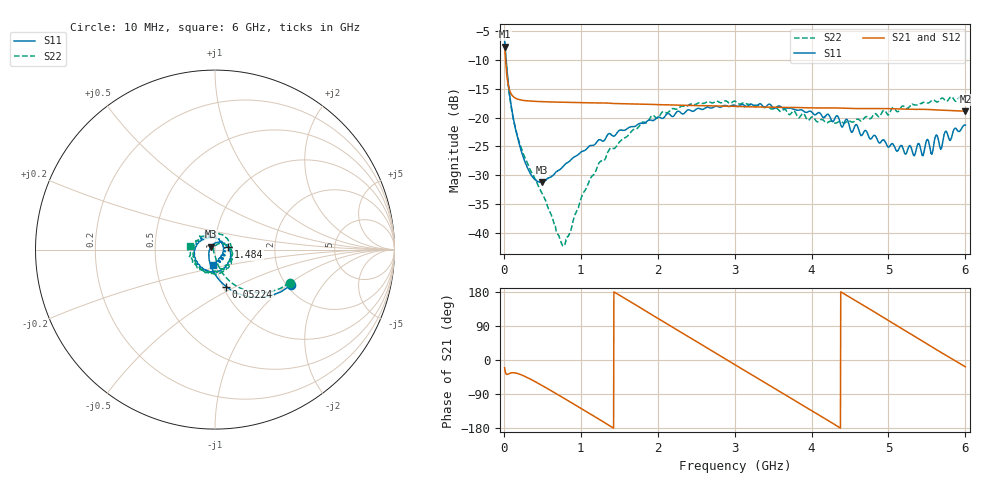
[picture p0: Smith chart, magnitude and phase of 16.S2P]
!Agilent Technologies,E5071C,MY46316741,A.11.02
!Date: Thu Jul 30 16:13:29 2020
!Data & Calibration Information:
!Freq	S11:SOLT4(ON)	S21:SOLT4(ON)	S12:SOLT4(ON)	S22:SOLT4(ON)
!PortZ  Port1:50+j0  Port2:50+j0
!Above PortZ is port z conversion or system Z0 setting when saving the data.
!When reading, reference impedance value at option line is always used.
# Hz S dB R 50
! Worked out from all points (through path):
!   1561 points, 10 MHz to 6 GHz, reference 50 ohm
!   highest |S21| = -7.68 dB at 10 MHz (marker M1); lowest = -18.9 dB at 6 GHz (marker M2)
!   group delay of S21, straight-line fit = 337 ps
!   lowest |S11| = -31.2 dB at 493.8 MHz (marker M3), VSWR 1.06, Z = 47.8 + j1.56 ohm
!   |S11| at or under -10 dB: 29.81 MHz to end of sweep
!   |S22| runs from -42.3 to -6.8 dB; largest |S21 - S12| = 0.0019
!   S11 on the Smith chart (normalised r, x): 10 MHz: 2.10, -1.07; 52.24 MHz: 1.03, -0.45; 1.484 GHz: 1.16, +0.03; 6 GHz: 0.96, -0.16
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1e7  -6.61 -25.1  -7.68 -20.5  -7.68 -20.5  -6.85 -23.9
5.223718e7  -13.35 -73.2  -13.96 -37.4  -13.96 -37.4  -13.71 -63.4
1.290321e8  -20.56 -104.1  -16.44 -33.7  -16.44 -33.7  -20.60 -77.9
2.442244e8  -26.56 -137.2  -17.01 -40.6  -17.01 -40.7  -26.01 -84.7
4.938077e8  -31.24 143.5  -17.24 -66.9  -17.24 -67.0  -33.11 -102.4
7.74109e8  -28.42 83.6  -17.34 -100.0  -17.34 -100.2  -42.35 172.5
1.012173e9  -25.93 55.0  -17.41 -128.9  -17.42 -129.0  -33.70 86.7
1.242558e9  -23.84 33.9  -17.47 -157.0  -17.47 -157.1  -27.79 57.4
1.484462e9  -22.45 10.4  -17.59 173.3  -17.59 173.0  -24.60 30.4
2.006667e9  -19.92 -27.9  -17.77 109.3  -17.76 109.2  -20.02 -21.8
3.005e9  -17.89 -103.7  -18.05 -12.5  -18.06 -13.0  -17.16 -126.8
3.534885e9  -18.32 -149.3  -18.22 -77.0  -18.21 -77.5  -18.34 170.2
4.007173e9  -19.11 173.2  -18.32 -134.4  -18.31 -135.1  -19.89 101.7
4.586974e9  -21.27 115.1  -18.44 154.9  -18.45 154.1  -20.32 6.4
5.001667e9  -25.11 57.7  -18.45 104.0  -18.45 103.2  -19.53 -58.2
5.443237e9  -26.50 -19.4  -18.58 49.8  -18.59 48.9  -17.39 -116.9
5.504673e9  -23.83 -31.3  -18.59 42.1  -18.59 41.3  -17.48 -124.2
5.562269e9  -26.36 -41.2  -18.63 34.9  -18.63 34.1  -17.05 -132.8
5.619865e9  -23.07 -51.7  -18.67 27.8  -18.67 27.0  -17.24 -138.1
5.681301e9  -25.53 -60.2  -18.72 20.3  -18.72 19.5  -16.72 -148.6
5.742737e9  -22.40 -68.9  -18.75 12.9  -18.75 12.1  -17.12 -153.7
6e9  -21.31 -99.3  -18.89 -18.0  -18.88 -18.9  -17.16 172.2
